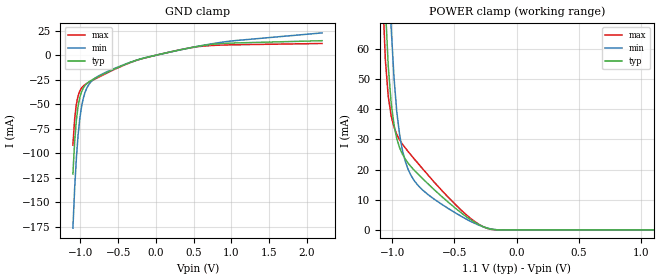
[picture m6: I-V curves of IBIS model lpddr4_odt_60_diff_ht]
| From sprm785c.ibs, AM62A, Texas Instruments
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|   Model lpddr4_odt_60_diff_ht
[Model] lpddr4_odt_60_diff_ht
Model_type Input
Polarity   Non-Inverting
Enable   Active-High
Vinl =  0.113V
Vinh =  0.253V
C_comp   2.516pF   2.456pF   2.551pF
[Model Spec]
Vinh   0.253V   0.247V   0.265V
Vinl   0.113V   0.107V   0.125V
[Temperature Range]   25.000   0.125k   -40.000
[Voltage Range]   1.100V   1.060V   1.170V
[C Comp Corner]
C_comp   2.516pF   2.456pF   2.551pF
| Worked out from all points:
|   GND clamp passes 1 mA (typ) near -0.05 V on its own axis
|   POWER clamp passes 1 mA (typ) near -0.27 V on its own axis
[GND_clamp]
|Voltage   I(typ)   I(min)   I(max)
-1.1V     -121.2mA   -176.5mA   -91.74mA
-1.077V   -88.47mA   -136.2mA   -65.3mA
-1.054V   -66.2mA    -104.8mA   -49.83mA
-1.031V   -51.88mA   -81.3mA    -41.24mA
-1.008V   -42.91mA   -64.3mA    -36.39mA
-985mV    -37.26mA   -52.3mA    -33.45mA
-940mV    -30.99mA   -37.97mA   -30.07mA
-825mV    -24.33mA   -24.6mA    -25.06mA
-252mV    -5.011mA   -4.993mA   -5.159mA
481mV     7.979mA    7.9mA      7.801mA
917mV     12.02mA    13.66mA    10.39mA
2.2V      14.74mA    22.71mA    11.91mA
[POWER_clamp]
|Voltage   I(typ)   I(min)   I(max)
-1.1V     153.2mA    238mA      119.3mA
-1.077V   105.7mA    174.3mA    78.85mA
-1.054V   74.17mA    126.4mA    56.33mA
-1.031V   54.35mA    91.72mA    44.31mA
-1.008V   42.29mA    67.4mA     37.87mA
-963mV    30.31mA    39.35mA    31.67mA
-940mV    27.23mA    31.63mA    29.86mA
-894mV    23.45mA    22.69mA    27.16mA
-848mV    20.95mA    18.03mA    24.8mA
-665mV    13.43mA    10.26mA    15.95mA
-206mV    235.7uA    300uA      179.3uA
1.1V      0A         0A         0A
